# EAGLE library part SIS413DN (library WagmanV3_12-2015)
MOSFET
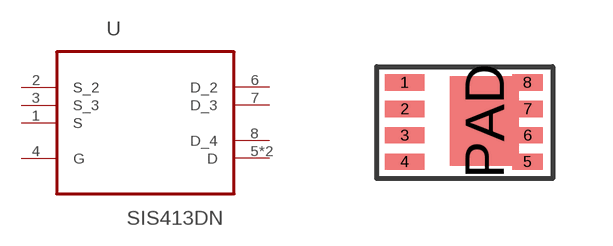
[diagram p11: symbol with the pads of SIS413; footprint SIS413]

Designator prefix U

## SIS413DN  [SIS413]
1  S  pas
2  S_2  pas
3  S_3  pas
4  G  pas
5  D  pas
6  D_2  pas
7  D_3  pas
8  D_4  pas
PAD  D  pas

## Footprint SIS413 (pad centres in mm)
smd 0.99 x 0.405: 1 0,0; 2 0,-0.66; 3 0,-1.32; 4 0,-1.98
smd 0.76 x 0.405: 5 3.075,-1.98; 6 3.075,-1.32; 7 3.075,-0.66; 8 3.075,0
smd 1.725 x 2.235: PAD 1.992,-0.96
